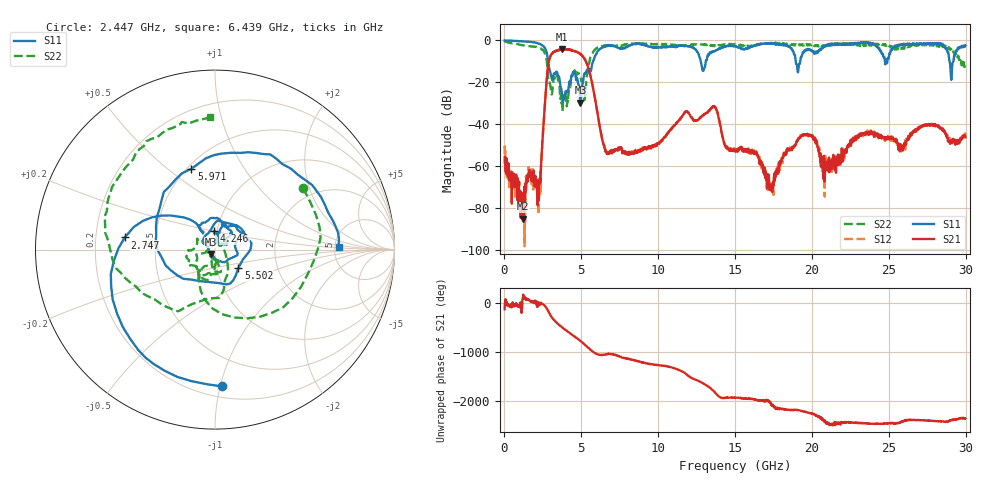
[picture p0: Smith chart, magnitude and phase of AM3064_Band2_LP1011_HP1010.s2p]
# Hz S DB R 50.0
!freq dBS11 angS11 dBS21 angS21 dBS12 angS12 dBS22 angS22
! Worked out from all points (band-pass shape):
!   1600 points, 10 MHz to 29.98 GHz, reference 50 ohm
!   highest |S21| = -4.19 dB at 3.759 GHz (marker M1); lowest = -85.2 dB at 1.228 GHz (marker M2)
!   |S21| within 3 dB of the highest: 3.01 GHz to 5.047 GHz (2.037 GHz wide, 50.6 % of centre)
!   lowest |S11| = -29.8 dB at 4.94 GHz (marker M3), VSWR 1.07, Z = 47.9 - j2.35 ohm
!   |S11| at or under -10 dB: 2.838 GHz to 5.763 GHz (2.925 GHz wide, 68 % of centre); 12.77 GHz to 13.1 GHz (326.5 MHz wide, 2.52 % of centre); 18.95 GHz to 19.24 GHz (295.2 MHz wide, 1.55 % of centre)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
!   |S22| runs from -33.7 to -0.2 dB; largest |S21 - S12| = 0.014
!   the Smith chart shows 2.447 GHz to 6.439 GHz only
!   S11 on the Smith chart (normalised r, x): 2.447 GHz: 0.28, -1.01; 2.747 GHz: 0.33, +0.06; 4.246 GHz: 0.97, +0.20; 5.502 GHz: 1.27, -0.27; 5.971 GHz: 0.53, +0.61; 6.439 GHz: 5.41, +0.33
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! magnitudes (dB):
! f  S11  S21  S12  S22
! 10 MHz  0.0  -55.7  -50.3  -0.2
! 1.228 GHz  -0.5  -85.2  -74.4  -2.4
! 1.678 GHz  -0.7  -63.8  -62.5  -2.9
! 2.184 GHz  -1.4  -68.7  -72.8  -3.4
! 2.447 GHz  -2.4  -51.5  -50.3  -4.5
! 2.747 GHz  -5.9  -18.9  -18.9  -9.7
! 3.759 GHz  -25.8  -4.2  -4.2  -32.1
! 4.246 GHz  -19.7  -4.4  -4.5  -22.3
! 4.94 GHz  -29.8  -6.5  -6.5  -17.0
! 5.015 GHz  -22.4  -7.1  -7.0  -19.6
! 5.502 GHz  -15.6  -14.3  -14.1  -11.2
! 5.971 GHz  -6.6  -31.2  -31.3  -3.8
! 6.439 GHz  -3.2  -49.6  -49.4  -2.6
! 10 GHz  -3.4  -49.1  -48.8  -1.9
! 13.6 GHz  -5.2  -31.9  -31.6  -2.6
! 15 GHz  -2.6  -53.1  -53.0  -1.9
! 17.37 GHz  -1.5  -69.9  -70.0  -1.2
! 19.99 GHz  -4.7  -45.9  -46.1  -1.9
! 20.82 GHz  -2.8  -67.5  -62.2  -2.3
! 25 GHz  -8.3  -46.5  -47.3  -2.2
! 29.08 GHz  -17.5  -48.3  -48.6  -5.2
! 29.98 GHz  -2.3  -46.4  -45.1  -10.3
